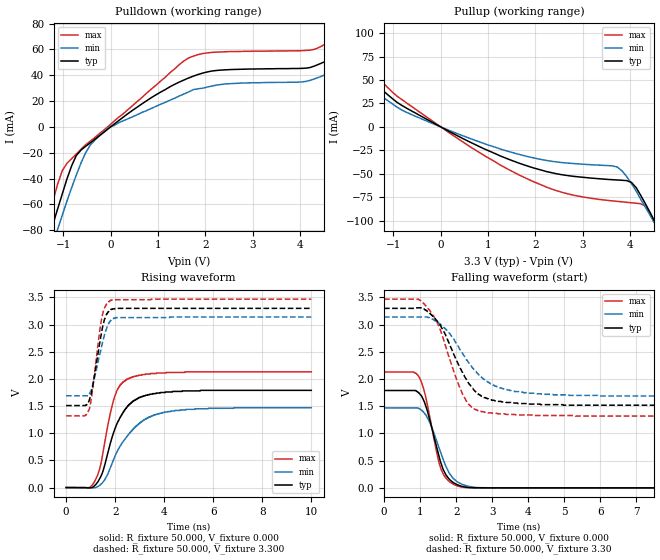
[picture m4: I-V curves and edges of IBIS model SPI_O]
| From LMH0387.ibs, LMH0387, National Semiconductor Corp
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|   Model SPI_O
[Model]  SPI_O
Model_type Output
Enable   Active-High
Vmeas =  1
C_comp   542.2fF   513.0fF   577.4fF
[Temperature Range]   25.0000   85.0000   -40.0000
[Voltage Range]   3.3000V   3.1350V   3.4650V
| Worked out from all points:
|   slope of the pulldown table from 0 to 0.495 V, typ, clamps not added: 36.3 ohm
|   slope of the pullup table from 0 to 0.495 V, typ, clamps not added: 37.7 ohm
|   rising waveform, R_fixture 50.000, V_fixture 0.000: 20-80 % time 859ps typ, 1.23ns min, 592ps max; typ from 0 V to 1.79 V
|   rising waveform, R_fixture 50.000, V_fixture 3.300: 20-80 % time 397ps typ, 455ps min, 358ps max; typ from 1.51 V to 3.3 V
|   falling waveform, R_fixture 50.000, V_fixture 0.000: 20-80 % time 434ps typ, 505ps min, 397ps max; typ from 1.79 V to 0 V
|   falling waveform, R_fixture 50.000, V_fixture 3.30: 20-80 % time 814ps typ, 1ns min, 685ps max; typ from 3.3 V to 1.51 V
[Pulldown]
|Voltage   I(typ)   I(min)   I(max)
-3.3V     -382mA     -355mA     -418mA
-1.42V    -101mA     -114mA     -86mA
-1.22V    -75.5mA    -90.7mA    -57.5mA
-1.02V    -51.7mA    -68.2mA    -33.7mA
-726mV    -22.2mA    -37.3mA    -21mA
-231mV    -6.67mA    -6.62mA    -5mA
1.65V     37.9mA     27.1mA     53.4mA
4.22V     46mA       36.1mA     59.4mA
4.82V     56.2mA     46.2mA     70.4mA
5.21V     77mA       65.9mA     89.6mA
5.41V     90.8mA     76.9mA     107mA
6.6V      175mA      144mA      213mA
[Pullup]
|Voltage   I(typ)   I(min)   I(max)
-3.3V     175mA      144mA      213mA
-2.61V    126mA      105mA      151mA
-2.31V    105mA      87.8mA     124mA
-2.11V    90.7mA     76.7mA     107mA
-1.72V    63.5mA     54.7mA     74mA
-924mV    26.2mA     21.1mA     32.8mA
1.95V     -43.6mA    -32.9mA    -58.2mA
3.73V     -56.6mA    -42.8mA    -79.4mA
4.13V     -64.8mA    -68.5mA    -81.4mA
4.32V     -81.6mA    -85.4mA    -84.4mA
4.62V     -111mA     -112mA     -114mA
6.6V      -384mA     -356mA     -421mA
[Ramp]
|variable   typ   min   max
dV/dt_r   1.0766/441.4p   882.33m/1.233n   1.2789/595.4p
dV/dt_f   1.0767/868.3p   882.83m/1.233n   1.2794/598.4p
R_load  = 50
[Rising Waveform]
R_fixture = 50.000
V_fixture = 0.000
V_fixture_min = 0.000
V_fixture_max = 0.000
|  time   V(typ)   V(min)   V(max)
0s        653pV      1.06nV     657pV
920ps     -5.39mV    -3.18mV    -3.57mV
1.15ns    28.9mV     -4.33mV    101mV
1.38ns    167mV      44mV       361mV
1.72ns    670mV      269mV      1.19V
1.97ns    1.05V      551mV      1.66V
2.5ns     1.49V      954mV      2V
3.18ns    1.69V      1.25V      2.08V
4.28ns    1.76V      1.41V      2.12V
10ns      1.79V      1.47V      2.13V
[Rising Waveform]
R_fixture = 50.000
V_fixture = 3.300
V_fixture_min = 3.1350
V_fixture_max = 3.4650
|  time   V(typ)   V(min)   V(max)
0s        1.51V      1.69V      1.32V
770ps     1.51V      1.69V      1.32V
950ps     1.62V      1.72V      1.45V
1.07ns    1.83V      1.86V      1.77V
1.31ns    2.49V      2.32V      2.67V
1.45ns    2.86V      2.6V       3.12V
1.61ns    3.15V      2.87V      3.35V
1.82ns    3.28V      3.08V      3.45V
2.02ns    3.3V       3.13V      3.46V
10ns      3.3V       3.14V      3.47V
[Falling Waveform]
R_fixture = 50.000
V_fixture = 0.000
V_fixture_min = 0.000
V_fixture_max = 0.000
|  time   V(typ)   V(min)   V(max)
0s        1.79V      1.47V      2.13V
820ps     1.79V      1.47V      2.13V
990ps     1.73V      1.45V      2.02V
1.21ns    1.4V       1.28V      1.5V
1.45ns    769mV      879mV      684mV
1.58ns    453mV      633mV      345mV
1.8ns     167mV      279mV      123mV
2.05ns    52.1mV     105mV      31.6mV
2.73ns    988uV      2.02mV     733uV
10ns      157nV      526nV      431nV
[Falling Waveform]
R_fixture = 50.000
V_fixture = 3.30
V_fixture_min = 3.1350
V_fixture_max = 3.4650
|  time   V(typ)   V(min)   V(max)
0s        3.3V       3.14V      3.47V
950ps     3.31V      3.14V      3.47V
1.2ns     3.25V      3.14V      3.32V
1.52ns    3.02V      3.03V      2.98V
1.81ns    2.65V      2.85V      2.39V
2.21ns    2.08V      2.44V      1.68V
2.64ns    1.71V      2.07V      1.41V
3.2ns     1.59V      1.84V      1.36V
3.97ns    1.54V      1.74V      1.34V
10ns      1.51V      1.69V      1.32V
